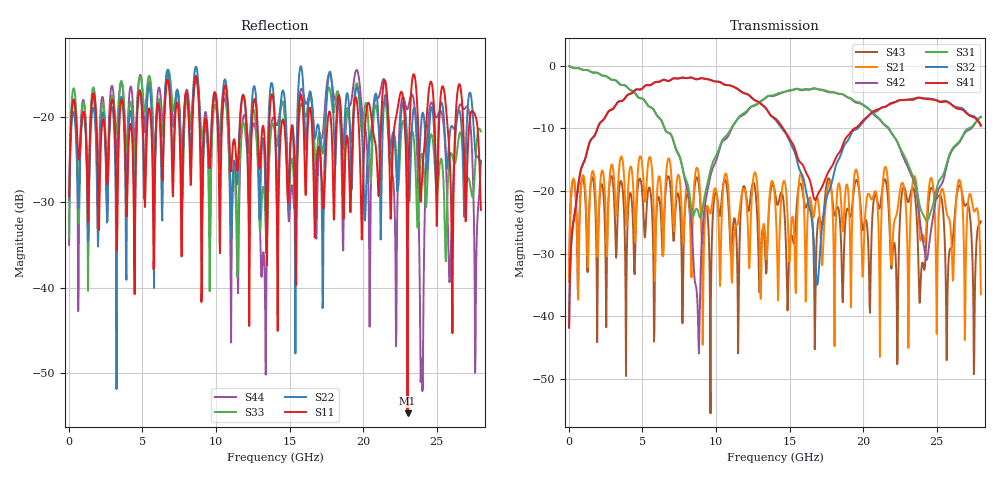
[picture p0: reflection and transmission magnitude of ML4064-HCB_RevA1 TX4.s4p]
! TOUCHSTONE file generated by CST DESIGN STUDIO
! Date and time: Wed Aug 26 10:54:20 2020
! Project name:  Project name: C:\Users\Simulation2\Temp\DE66\Untitled_0.cst
! Tree item: Tasks\SPara1\S-Parameters
# GHz S MA R 50
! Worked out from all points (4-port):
!   1000 points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, 28 MHz to 28 GHz, reference 50 ohm
!   strongest paths, dB at 28 MHz, 7.028 GHz, 14.03 GHz, 21.03 GHz, 28 GHz:
!     S41: -41.8, -2.1, -8.4, -6.9, -9.6
!     S32: -41.8, -2.1, -8.6, -7.1, -9.4
!     S31: -0.1, -11.4, -4.6, -8.3, -8.2
!     S42: -0.1, -11.4, -4.7, -8.4, -8.2
!     S21: -34.5, -19.9, -21.7, -24.6, -36.5
!     S43: -34.0, -23.8, -20.5, -22.4, -24.8
!   lowest |S11| = -54.7 dB at 23.02 GHz (marker M1), VSWR 1.00, Z = 50.1 + j0.126 ohm
!   |S11| at or under -10 dB: start of sweep to end of sweep
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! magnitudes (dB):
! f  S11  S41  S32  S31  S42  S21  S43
! 28 MHz  -29.3  -41.8  -41.8  -0.1  -0.1  -34.5  -34.0
! 8.792 GHz  -17.0  -2.1  -2.1  -23.3  -41.3  -16.8  -18.3
! 16.88 GHz  -24.7  -20.8  -35.0  -3.7  -3.7  -21.1  -26.2
! 23.02 GHz  -54.7  -5.4  -5.4  -15.5  -16.1  -30.1  -21.6
! 23.97 GHz  -28.4  -5.1  -5.2  -23.3  -26.7  -27.4  -32.2
! 24.58 GHz  -15.9  -5.4  -5.3  -23.4  -26.7  -18.0  -19.7
! 28 GHz  -30.9  -9.6  -9.4  -8.2  -8.2  -36.5  -24.8
